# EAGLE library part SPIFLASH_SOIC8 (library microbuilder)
SOIC8 SPI Flash Be careful with the size since SOIC8 flash comes in several 'widths' SOIC8 150 mil M25P16 - 16Mbit (2Mbit x 8) Serial Flash (75MHz SPI Bus), Supply: 2.7-3.6V Digikey: SOIC8 - M25P16-VMN6P-ND SOIC8 208 mil W25Q16BVSSIG - 16Mbit (2Mbit x 8) Serial Flash (104MHz SPI Bus), Supply: 2.7-3.6V Digikey: SOIC8 - W25Q16BVSSIG-ND
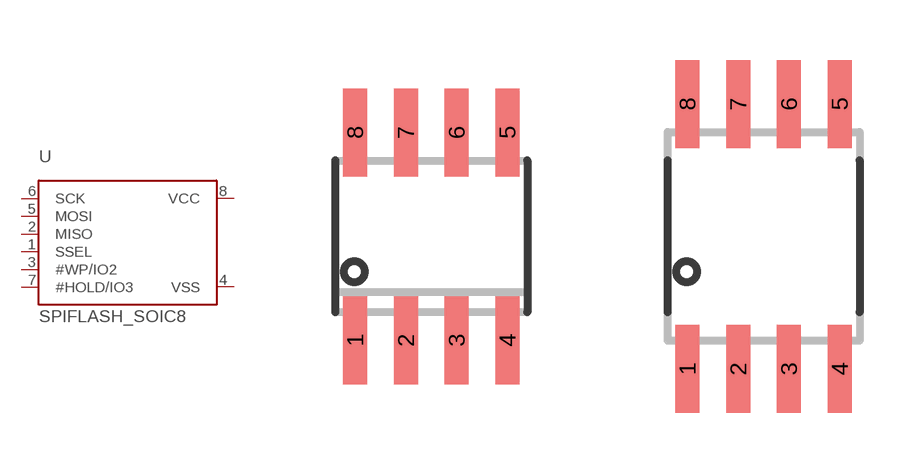
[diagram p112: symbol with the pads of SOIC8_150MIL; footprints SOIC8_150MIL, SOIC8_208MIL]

Designator prefix U

## SPIFLASH_SOIC8  [SOIC8_150MIL]
1  SSEL
2  MISO
3  #WP/IO2
4  VSS
5  MOSI
6  SCK
7  #HOLD/IO3
8  VCC

## SPIFLASH_SOIC8208MIL  [SOIC8_208MIL]
Pads as for SOIC8_150MIL

## Footprint SOIC8_150MIL (pad centres in mm)
Small Outline IC - 150mil Wide
smd 0.6 x 2.2: 1 -1.905,-2.6; 2 -0.635,-2.6; 3 0.635,-2.6; 4 1.905,-2.6; 5 1.905,2.6; 6 0.635,2.6; 7 -0.635,2.6; 8 -1.905,2.6

## Footprint SOIC8_208MIL (pad centres in mm)
Small Outline IC - 208mil Wide
smd 0.6 x 2.2: 1 -1.905,-3.315; 2 -0.635,-3.315; 3 0.635,-3.315; 4 1.905,-3.315; 5 1.905,3.315; 6 0.635,3.315; 7 -0.635,3.315; 8 -1.905,3.315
